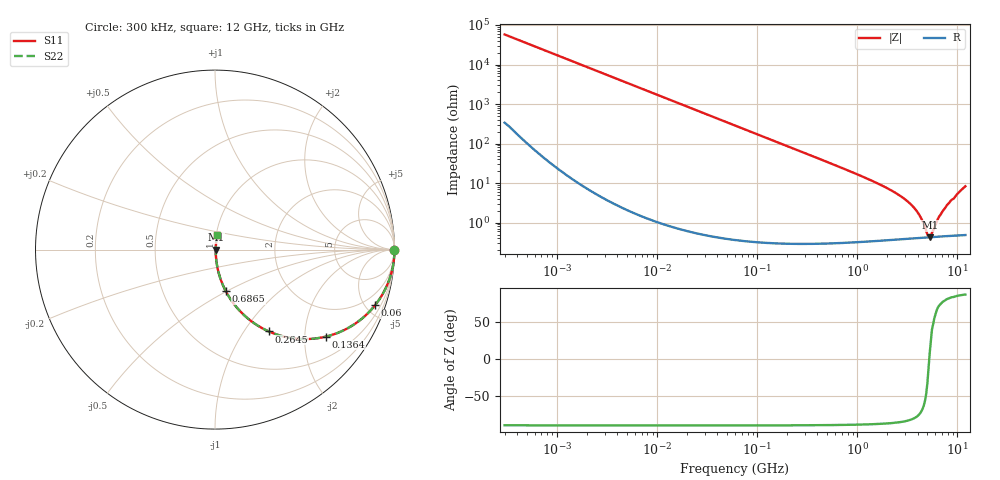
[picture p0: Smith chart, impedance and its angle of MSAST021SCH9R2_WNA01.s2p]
! MSAST021SCH9R2_WNA01  S-PARAMETER MODEL  ( General Type )
! Model Generated by TAIYO YUDEN Corporation (http://www.ty-top.com)
! Version 2.0
! TAIYO YUDEN Control No. 181101
! Copyright(c) 2015 TAIYO YUDEN CO.,LTD. All Rights Reserved.
! Product Description (link to TY-COMPAS)
! https://ds.yuden.co.jp/TYCOMPAS/or/detail?pn=MSAST021SCH9R2CWNA01&u=M
! Products Name : Multilayer Ceramic Capacitors
! Characteristics :
!  Capacitance : 9.2 pF , Rated Voltage : 25V , TCC : CH / C0H
!  Case Size : 0.25 x 0.125 / 0.0098 x 0.0049 [mm/inch] , Thickness : 0.125 / 0.0049 [mm/inch]
!  (Conditions: Temperature = 25 degC , DC Bias Current/Voltage = 0A / 0V)
! External Node Assignments :
!  1  o---| |---o  2
! GND o---------o GND
! Frequency Range : 0.3MHz  -  12000MHz  [ 401 STEP ]
# MHz S RI R 50
! Freq[MHz].  S11 Real  S11 Imag  S21 Real  S21 Imag  S12 Real  S12 Imag  S22 Real  S22 Imag
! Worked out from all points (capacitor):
!   401 points, 300 kHz to 12 GHz, reference 50 ohm
!   read as one part in series: C = 9.2 pF near 316.3 kHz
!   lowest |Z| = 431 mohm at 5.279 GHz (marker M1)
!   series resonance near 5.23 GHz, so ESL is about 100 pH
!   S11 on the Smith chart (normalised r, x): 300 kHz: open; 60 MHz: 1.01, -5.77; 136.4 MHz: 1.01, -2.53; 264.5 MHz: 1.01, -1.30; 686.5 MHz: 1.01, -0.50; 12 GHz: 1.01, +0.17
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0.3  1 -0.00173  1.32e-05 0.00173  1.32e-05 0.00173  1 -0.00173
1.769972  0.9999 -0.0102  0.000114 0.0102  0.000114 0.0102  0.9999 -0.0102
10.44266  0.9963 -0.0601  0.00367 0.0601  0.00367 0.0601  0.9963 -0.0601
26.39317  0.9771 -0.1491  0.0229 0.1491  0.0229 0.1491  0.9771 -0.1491
60  0.8923 -0.3094  0.1077 0.3094  0.1077 0.3094  0.8923 -0.3094
89.27472  0.7892 -0.407  0.2108 0.407  0.2108 0.407  0.7892 -0.407
136.3989  0.6161 -0.4851  0.3839 0.4851  0.3839 0.4851  0.6161 -0.4851
264.5085  0.2993 -0.4558  0.7007 0.4558  0.7007 0.4558  0.2993 -0.4558
353.9943  0.1928 -0.3915  0.8072 0.3915  0.8072 0.3915  0.1928 -0.3915
686.4755  0.0603 -0.232  0.9397 0.232  0.9397 0.232  0.0603 -0.232
2088.533  0.00837 -0.0687  0.9916 0.0687  0.9916 0.0687  0.00837 -0.0687
2870.14  0.00556 -0.0416  0.9944 0.0416  0.9944 0.0416  0.00556 -0.0416
3642.919  0.00457 -0.0241  0.9954 0.0241  0.9954 0.0241  0.00457 -0.0241
4158.869  0.00431 -0.015  0.9957 0.015  0.9957 0.015  0.00431 -0.015
4502.883  0.00424 -0.00973  0.9958 0.00973  0.9958 0.00973  0.00424 -0.00973
5006.236  0.00423 -0.00272  0.9958 0.00272  0.9958 0.00272  0.00423 -0.00272
5278.635  0.00426 0.000534  0.9957 -0.000534  0.9957 -0.000534  0.00426 0.000534
5565.855  0.00431 0.00355  0.9957 -0.00355  0.9957 -0.00355  0.00431 0.00355
6524.734  0.00459 0.013  0.9954 -0.013  0.9954 -0.013  0.00459 0.013
7448.838  0.005 0.022  0.995 -0.022  0.995 -0.022  0.005 0.022
10236.47  0.0079 0.0561  0.9921 -0.0561  0.9921 -0.0561  0.0079 0.0561
12000  0.0116 0.0817  0.9884 -0.0817  0.9884 -0.0817  0.0116 0.0817
